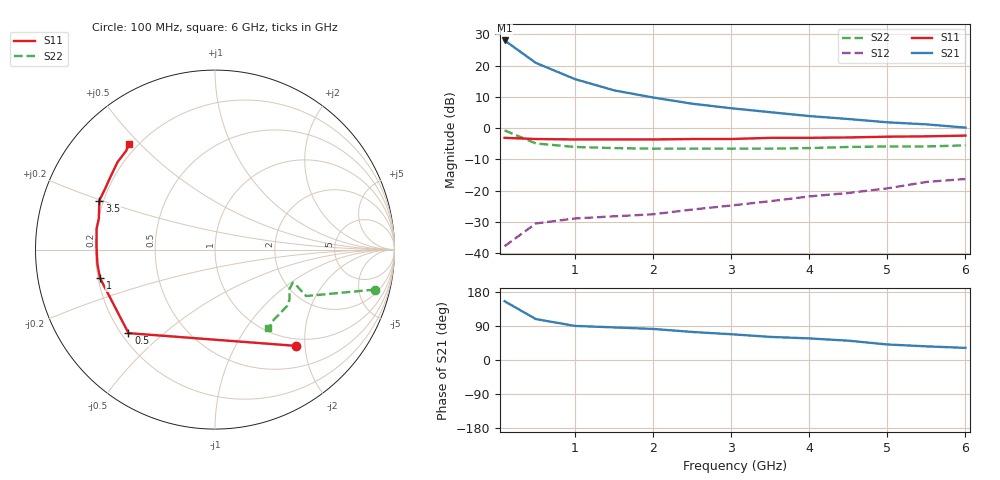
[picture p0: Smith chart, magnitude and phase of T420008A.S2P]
!AT-42000
!S-PARAMETERS at Vce=8V  Ic=10mA.  LAST UPDATED 07-21-92
# ghz s ma r 50
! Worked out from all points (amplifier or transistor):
!   13 points, 100 MHz to 6 GHz, reference 50 ohm
!   highest |S21| = 28.0 dB at 100 MHz (marker M1)
!   |S21| within 3 dB of that: start of sweep to 267.5 MHz
!   unconditionally stable (mu >= 1): 1.285 GHz to 5.047 GHz
!   at 1 GHz: K = 0.80, MSG = 22.3 dB, |S12| = -28.9 dB
!   at 3 GHz: K = 1.52, MAG = 11.3 dB, |S12| = -24.7 dB
!   at 6 GHz: K = 0.77, MSG = 8.2 dB, |S12| = -16.2 dB
!   lowest NFmin = 1.00 dB at 100 MHz
!   S11 on the Smith chart (normalised r, x): 100 MHz: 0.86, -1.82; 500 MHz: 0.23, -0.39; 1 GHz: 0.21, -0.12; 3.5 GHz: 0.18, +0.20; 6 GHz: 0.17, +0.47
0.1  0.7 -50.0  25.19 155.0  0.013 71.0  0.92 -14.0
0.5  0.67 -136.0  11.04 108.0  0.03 43.0  0.57 -27.0
1  0.66 -166.0  6.08 90.0  0.036 47.0  0.5 -24.0
1.5  0.66 -173.0  4.02 86.0  0.039 52.0  0.48 -23.0
2  0.66 179.0  3.09 82.0  0.042 57.0  0.47 -23.0
2.5  0.67 170.0  2.46 74.0  0.05 66.0  0.47 -23.0
3  0.67 165.0  2.08 68.0  0.058 72.0  0.47 -26.0
3.5  0.7 157.0  1.8 61.0  0.068 77.0  0.47 -28.0
4  0.7 151.0  1.56 57.0  0.081 82.0  0.48 -30.0
4.5  0.71 145.0  1.4 51.0  0.092 86.0  0.5 -34.0
5  0.73 138.0  1.24 41.0  0.109 87.0  0.51 -38.0
5.5  0.74 132.0  1.15 36.0  0.138 88.0  0.51 -50.0
6  0.76 129.0  1.02 32.0  0.154 87.0  0.53 -56.0
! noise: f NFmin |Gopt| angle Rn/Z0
0.1  1  0.04  13  0.13
0.5  1.1  0.05  69  0.13
1  1.5  0.09  127  0.12
2  1.9  0.23  171  0.11
4  3  0.47  -154  0.14
